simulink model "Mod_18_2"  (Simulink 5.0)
settings: Solver=ode45  StartTime=0.0  StopTime=400  MaxStep=0.005  RelTol=1e-3
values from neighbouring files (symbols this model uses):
  Cp = 7620    [Dados_18_2.m]
  KT_Te = 1    [Dados_18_2.m]
  KT_We = -185.52    [Dados_18_2.m]
  KT_Wv = 5614.1    [Dados_18_2.m]
  m = 3.5    [Dados_18_2.m]
  T0 = Tbarra    (= 30.276)    [Dados_18_2.m]
  Tal = 70    [Dados_18_2.m]
  Tbarra = 30.276    [Dados_18_2.m]
  Tebarra = 21    [Dados_18_2.m]
  Tebarra_deg = Tebarra    [Graf_18_2.m]
  Webarra = 0.05    [Dados_18_2.m]
  Webarra_deg = Webarra    [Graf_18_2.m]
  Wvbarra = 1.6524e-3    (= 0.0016524)    [Dados_18_2.m]
  Wvbarra_deg = Wvbarra    [Graf_18_2.m]

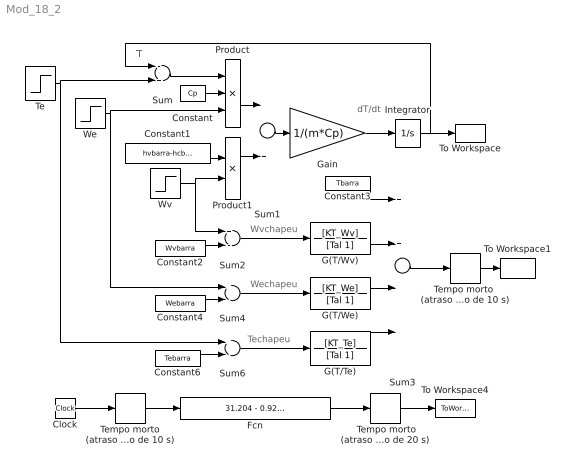
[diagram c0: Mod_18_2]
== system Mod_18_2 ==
  note: T
  note: dT/dt
  note: Wvchapeu
  note: Wechapeu
  note: Techapeu
  " Tempo morto (atraso puro de 20 s)" : TransportDelay  DelayTime=20  InitialInput=T0  BufferSize=4096
  Clock : Clock
  Constant : Constant  Value=Cp
  Constant1 : Constant  Value=hvbarra-hcbarra
  Constant2 : Constant  Value=Wvbarra
  Constant3 : Constant  Value=Tbarra
  Constant4 : Constant  Value=Webarra
  Constant6 : Constant  Value=Tebarra
  Fcn : Fcn  Expr=31.204 - 0.92767*exp(-u/70)
  G(T/Te) : TransferFcn  Numerator=[KT_Te]  Denominator=[Tal 1]
  G(T/We) : TransferFcn  Numerator=[KT_We]  Denominator=[Tal 1]
  G(T/Wv) : TransferFcn  Numerator=[KT_Wv]  Denominator=[Tal 1]
  Gain : Gain  Gain=1/(m*Cp)
  Integrator : Integrator  InitialCondition=T0
  Product : Product  Inputs=3
  Product1 : Product
  Sum : Sum  Inputs=-+
  Sum1 : Sum
  Sum2 : Sum  Inputs=+-
  Sum3 : Sum  Inputs=4
  Sum4 : Sum  Inputs=+-
  Sum6 : Sum  Inputs=+-
  Te : Step  Time=10  Before=Tebarra  After=Tebarra_deg  SampleTime=0
  Tempo morto (atraso puro de 10 s) : TransportDelay  DelayTime=10  BufferSize=4096
  Tempo morto  (atraso puro de 10 s) : TransportDelay  DelayTime=10  InitialInput=T0  BufferSize=4096
  To Workspace : ToWorkspace  VariableName=T_nl  SampleTime=-1  SaveFormat=Array
  To Workspace1 : ToWorkspace  VariableName=T_lin  SampleTime=-1  SaveFormat=Array
  To Workspace4 : ToWorkspace  VariableName=T_lin1  SampleTime=-1  SaveFormat=Array
  We : Step  Time=10  Before=Webarra  After=Webarra_deg  SampleTime=0
  Wv : Step  Time=10  Before=Wvbarra  After=Wvbarra_deg  SampleTime=0
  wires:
  Te/1 -> Sum/2, Sum6/1
  Sum/1 -> Product/1
  Constant/1 -> Product/2
  We/1 -> Product/3, Sum4/1
  Product/1 -> Sum1/1
  Product1/1 -> Sum1/2
  Constant1/1 -> Product1/1
  Sum1/1 -> Gain/1
  Gain/1 -> Integrator/1
  Integrator/1 -> Sum/1, To Workspace/1
  Wv/1 -> Product1/2, Sum2/1
  Sum2/1 -> G(T/Wv)/1
  Constant2/1 -> Sum2/2
  G(T/Wv)/1 -> Sum3/2
  Constant3/1 -> Sum3/1
  Sum3/1 -> Tempo morto  (atraso puro de 10 s)/1
  Constant4/1 -> Sum4/2
  Sum4/1 -> G(T/We)/1
  Constant6/1 -> Sum6/2
  Sum6/1 -> G(T/Te)/1
  G(T/Te)/1 -> Sum3/4
  Clock/1 -> Tempo morto (atraso puro de 10 s)/1
  Fcn/1 -> " Tempo morto (atraso puro de 20 s)"/1
  Tempo morto (atraso puro de 10 s)/1 -> Fcn/1
  G(T/We)/1 -> Sum3/3
  " Tempo morto (atraso puro de 20 s)"/1 -> To Workspace4/1
  Tempo morto  (atraso puro de 10 s)/1 -> To Workspace1/1
